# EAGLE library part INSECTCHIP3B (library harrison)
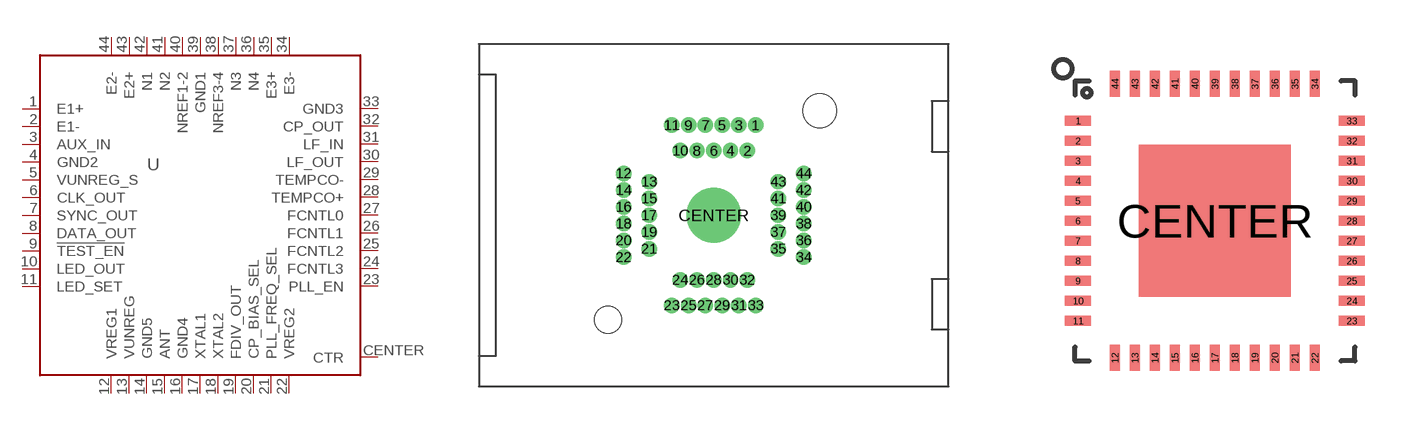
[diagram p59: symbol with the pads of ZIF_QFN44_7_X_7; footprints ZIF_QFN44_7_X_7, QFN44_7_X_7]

Designator prefix U

## INSECTCHIP3B_ZIF  [ZIF_QFN44_7_X_7]
1  E1+  in
2  E1-  in
3  AUX_IN  in
4  GND2  pwr
5  VUNREG_S  pwr
6  CLK_OUT  out
7  SYNC_OUT  out
8  DATA_OUT  out
9  !TEST_EN!  in
10  LED_OUT  pas
11  LED_SET  pas
12  VREG1  pwr
13  VUNREG  pwr
14  GND5  pwr
15  ANT  pas
16  GND4  pwr
17  XTAL1  pas
18  XTAL2  pas
19  FDIV_OUT  out
20  CP_BIAS_SEL  in
21  PLL_FREQ_SEL  in
22  VREG2  pwr
23  PLL_EN  in
24  FCNTL3  in
25  FCNTL2  in
26  FCNTL1  in
27  FCNTL0  in
28  TEMPCO+  pas
29  TEMPCO-  pas
30  LF_OUT  pas
31  LF_IN  pas
32  CP_OUT  pas
33  GND3  pwr
34  E3-  in
35  E3+  in
36  N4  in
37  N3  in
38  NREF3-4  in
39  GND1  pwr
40  NREF1-2  in
41  N2  in
42  N1  in
43  E2+  in
44  E2-  in
CENTER  CTR  pwr

## INSECTCHIP3B_QFN  [QFN44_7_X_7]
Pads as for ZIF_QFN44_7_X_7

## Footprint ZIF_QFN44_7_X_7 (pad centres in mm)
drill 0.41 pad 0.813: 1 2.5,5.37; 2 2,3.85; 3 1.5,5.37; 4 1,3.85; 5 0.5,5.37; 6 0,3.85; 7 -0.5,5.37; 8 -1,3.85; 9 -1.5,5.37; 10 -2,3.85; 11 -2.5,5.37; 12 -5.37,2.5; 13 -3.85,2; 14 -5.37,1.5; 15 -3.85,1; 16 -5.37,0.5; 17 -3.85,0; 18 -5.37,-0.5; 19 -3.85,-1; 20 -5.37,-1.5; 21 -3.85,-2; 22 -5.37,-2.5; 23 -2.5,-5.37; 24 -2,-3.85; 25 -1.5,-5.37; 26 -1,-3.85; 27 -0.5,-5.37; 28 0,-3.85; 29 0.5,-5.37; 30 1,-3.85; 31 1.5,-5.37; 32 2,-3.85; 33 2.5,-5.37; 34 5.37,-2.5; 35 3.85,-2; 36 5.37,-1.5; 37 3.85,-1; 38 5.37,-0.5; 39 3.85,0; 40 5.37,0.5; 41 3.85,1; 42 5.37,1.5; 43 3.85,2; 44 5.37,2.5
drill 2.26 pad 2.9: CENTER 0,0
hole 1.6 at -6.31,-6.23
hole 2 at 6.31,6.23

## Footprint QFN44_7_X_7 (pad centres in mm)
smd 0.65 x 0.25: 1 -3.425,2.5; 2 -3.425,2; 3 -3.425,1.5; 4 -3.425,1; 5 -3.425,0.5; 6 -3.425,0; 7 -3.425,-0.5; 8 -3.425,-1; 9 -3.425,-1.5; 10 -3.425,-2; 11 -3.425,-2.5; 23 3.425,-2.5; 24 3.425,-2; 25 3.425,-1.5; 26 3.425,-1; 27 3.425,-0.5; 28 3.425,0; 29 3.425,0.5; 30 3.425,1; 31 3.425,1.5; 32 3.425,2; 33 3.425,2.5
smd 0.25 x 0.65: 12 -2.5,-3.425; 13 -2,-3.425; 14 -1.5,-3.425; 15 -1,-3.425; 16 -0.5,-3.425; 17 0,-3.425; 18 0.5,-3.425; 19 1,-3.425; 20 1.5,-3.425; 21 2,-3.425; 22 2.5,-3.425; 34 2.5,3.425; 35 2,3.425; 36 1.5,3.425; 37 1,3.425; 38 0.5,3.425; 39 0,3.425; 40 -0.5,3.425; 41 -1,3.425; 42 -1.5,3.425; 43 -2,3.425; 44 -2.5,3.425
smd 3.8 x 3.8: CENTER 0,0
